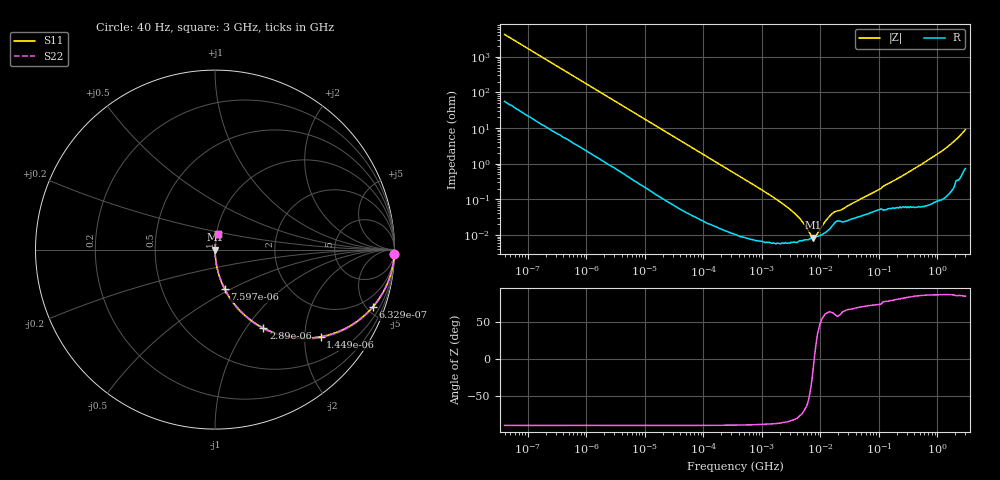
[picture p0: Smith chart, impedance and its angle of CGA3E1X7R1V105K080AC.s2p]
! S-parameter Generated by TDK Corporation
! Copyright(C) 2015 TDK Corporation.
! All Rights Reserved.
! TDK P/N: CGA3E1X7R1V105K080AC (Multilayer Ceramic Chip Capacitors)
! Property: C=1uF
! Size(LxWxT): 1.6x0.8x0.8mm, 0.063x0.031x0.031inches
! Model Type: s2p (Touchstone File Format Version 1.0)
! Frequency: DC=Yes Start=0.00004MHz Stop=3000MHz 396points Log-sweep
! Note: This model was converted from impedance.
! Model Generated on Jun. 23, 2015
! Hash(MD5):
! Port Assignments:
!  1 ---| |--- 2
! Applicable Conditions:
!  Temperature = 25 degC
!  DC Bias Voltage = 0 V
!  Small Signal Operation
! Terms and conditions regarding TDK Simulation Models
! (1)This simulation model is being provided solely for informational purposes. Please refer to the specifications of the products in terms of detailed characteristics of such products.
! (2)In no event shall TDK Corporation of any of its subsidiaries be liable for any loss or damage arising, directly or indirectly,
!  From any information contained in this simulation model, including, but not limited to loss or damages arising from any inaccuracies, omissions or errors in connection with such information.
! (3)Any and all copyrights on this simulation model are owned by TDK Corporation.
!  Duplication or redistribution of this simulation model without prior written permission from TDK Corporation is prohibited.
! (4)This simulation model is subject to any modification or change without any prior notice.
! (5)Neither TDK Corporation nor any of its subsidiaries shall make any warranty, express or implied,
!  Including but not limited to the correctness, implied warranties of merchantability and fitness for a particular purpose with respect to this simulation models.
! (6)The use of this simulation model shall be deemed to have consented to the terms and conditions hereof.
# MHz S MA R 50
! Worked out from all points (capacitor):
!   395 points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, 40 Hz to 3 GHz, reference 50 ohm
!   read as one part in series: C = 940 nF near 41.88 Hz
!   lowest |Z| = 8.43 mohm at 7.564 MHz (marker M1)
!   series resonance near 7.807 MHz, so ESL is about 440 pH
!   S11 on the Smith chart (normalised r, x): 40 Hz: 2, -85; 632.9 Hz: 1.07, -5.45; 1.449 kHz: 1.03, -2.40; 2.89 kHz: 1.02, -1.21; 7.597 kHz: 1.01, -0.47; 3 GHz: 1.01, +0.18
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4e-05  0.9994 -1.4  0.02364 87.9  0.02364 87.9  0.9994 -1.4
0.0001912643  0.9924 -6.4  0.1109 82.9  0.1109 82.9  0.9924 -6.4
0.0006328604  0.9349 -20.0  0.3428 69.2  0.3428 69.2  0.9349 -20.0
0.000834128  0.8961 -25.6  0.4323 63.6  0.4323 63.6  0.8961 -25.6
0.001449046  0.7629 -39.5  0.6367 49.7  0.6367 49.7  0.7629 -39.5
0.002889976  0.5143 -58.3  0.851 30.9  0.851 30.9  0.5143 -58.3
0.007596806  0.2259 -76.2  0.9714 13.1  0.9714 13.1  0.2259 -76.2
0.01739424  0.1021 -83.5  0.9936 5.9  0.9936 5.9  0.1021 -83.5
0.3464102  0.005305 -88.6  0.9999 0.3  0.9999 0.3  0.005305 -88.6
2.877491  0.0005584 -83.9  0.9999 0.0  0.9999 0.0  0.0005584 -83.9
4.354128  0.0003004 -76.8  0.9999 0.0  0.9999 0.0  0.0003004 -76.8
6.898837  9.877e-05 -36.3  0.9999 0.0  0.9999 0.0  9.877e-05 -36.3
7.22376  8.892e-05 -25.1  0.9999 0.0  0.9999 0.0  8.892e-05 -25.1
7.563987  8.43e-05 -9.9  0.9999 0.0  0.9999 0.0  8.43e-05 -9.9
8.683867  0.0001032 29.0  0.9999 -0.0  0.9999 -0.0  0.0001032 29.0
11.98465  0.000237 61.1  0.9999 -0.0  0.9999 -0.0  0.000237 61.1
17.31909  0.0004445 61.3  0.9998 -0.0  0.9998 -0.0  0.0004445 61.3
22.82706  0.0005081 62.3  0.9998 -0.0  0.9998 -0.0  0.0005081 62.3
150.6385  0.002852 78.8  0.9994 -0.2  0.9994 -0.2  0.002852 78.8
1141.26  0.02158 86.2  0.9988 -1.2  0.9988 -1.2  0.02158 86.2
2173.747  0.05047 83.3  0.9953 -2.9  0.9953 -2.9  0.05047 83.3
3000  0.08904 80.2  0.9888 -5.1  0.9888 -5.1  0.08904 80.2
